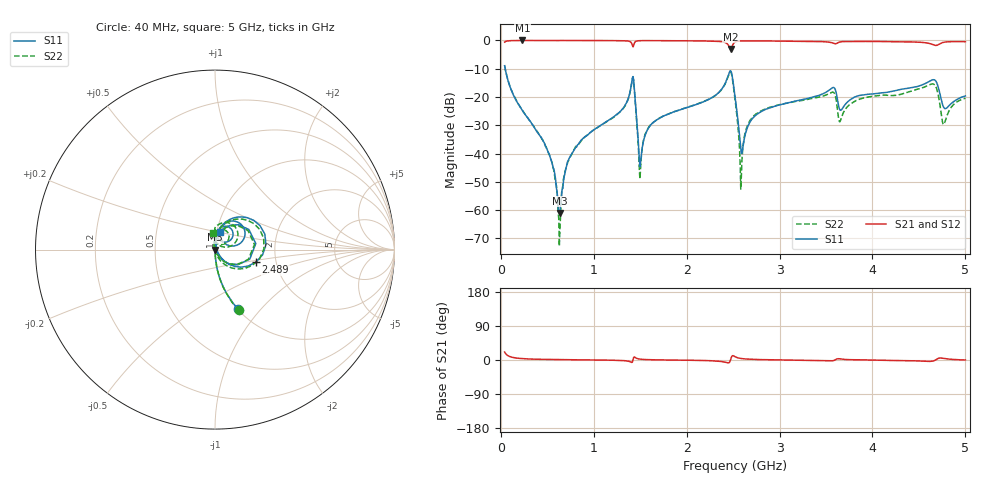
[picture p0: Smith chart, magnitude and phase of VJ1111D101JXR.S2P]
! VJ1111D101JXR
! DATE 02/15/2022  13:09
! CAPACITORS MOUNTED IN SERIES ON 25 MIL THICK MICROSTRIP SUBSTRATE
# GHz  S  MA  R  50.00
!  FREQ  S11M  S11A  S21M  S21A  S12M  S12A  S22M  S22A
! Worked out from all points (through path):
!   801 points, 40 MHz to 5 GHz, reference 50 ohm
!   highest |S21| = -0.01 dB at 232.2 MHz (marker M1); lowest = -3.0 dB at 2.477 GHz (marker M2)
!   lowest |S11| = -61.0 dB at 635.2 MHz (marker M3), VSWR 1.00, Z = 50.1 + j0.0249 ohm
!   |S11| at or under -10 dB: 45.93 MHz to end of sweep
!   |S22| runs from -72.7 to -8.8 dB; largest |S21 - S12| = 0.0096
!   S11 on the Smith chart (normalised r, x): 40 MHz: 1.00, -0.77; 2.489 GHz: 1.57, -0.23; 5 GHz: 1.04, +0.21
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0.04  0.3574 -68.8  0.9341 21.0  0.9335 21.1  0.362 -68.7
0.2322  0.05717 -86.3  0.9987 3.6  0.9981 3.6  0.05792 -86.6
0.5236  0.009267 -84.7  0.9968 1.4  1.001 1.4  0.009376 -85.2
0.6352  0.0008936 16.1  0.9968 0.9  0.9997 0.9  0.0004322 51.2
0.7096  0.006257 81.1  0.9965 0.7  0.9996 0.7  0.006435 85.9
0.8708  0.01748 85.4  0.9948 0.4  0.9994 0.3  0.01736 88.2
1.2924  0.05728 83.2  0.9883 -1.2  0.9929 -1.3  0.05635 84.0
1.4102  0.1906 46.6  0.8703 -6.4  0.8747 -6.5  0.185 45.9
1.5032  0.006714 40.5  0.9887 2.1  0.9959 2.0  0.005303 62.4
1.6954  0.04105 86.3  0.9901 0.3  0.9945 0.2  0.04134 89.1
2.4766  0.2854 5.7  0.7094 3.9  0.7126 3.8  0.2726 0.8
2.489  0.2385 -17.1  0.7811 10.7  0.7846 10.5  0.2256 -23.1
2.52  0.1026 -47.7  0.9354 8.8  0.9405 8.7  0.09256 -58.3
2.5882  0.01012 2.7  0.9789 3.9  0.9861 3.8  0.003927 135.3
2.737  0.04675 84.4  0.982 1.5  0.9868 1.3  0.04874 97.5
3.3508  0.09916 81.4  0.9625 -0.8  0.9672 -1.0  0.09459 88.6
3.574  0.1467 59.4  0.8975 -1.8  0.9025 -2.0  0.1221 61.9
3.6546  0.05822 55.6  0.9418 2.8  0.9489 2.6  0.03814 77.4
4.1754  0.1227 76.5  0.9525 -1.1  0.9595 -1.2  0.1067 88.2
4.6528  0.2024 44.3  0.8395 -2.7  0.8448 -2.9  0.1701 51.3
4.7706  0.06414 32.6  0.9298 4.1  0.9346 3.9  0.03304 62.9
5  0.1042 74.5  0.9498 0.1  0.9546 -0.2  0.0952 95.1
